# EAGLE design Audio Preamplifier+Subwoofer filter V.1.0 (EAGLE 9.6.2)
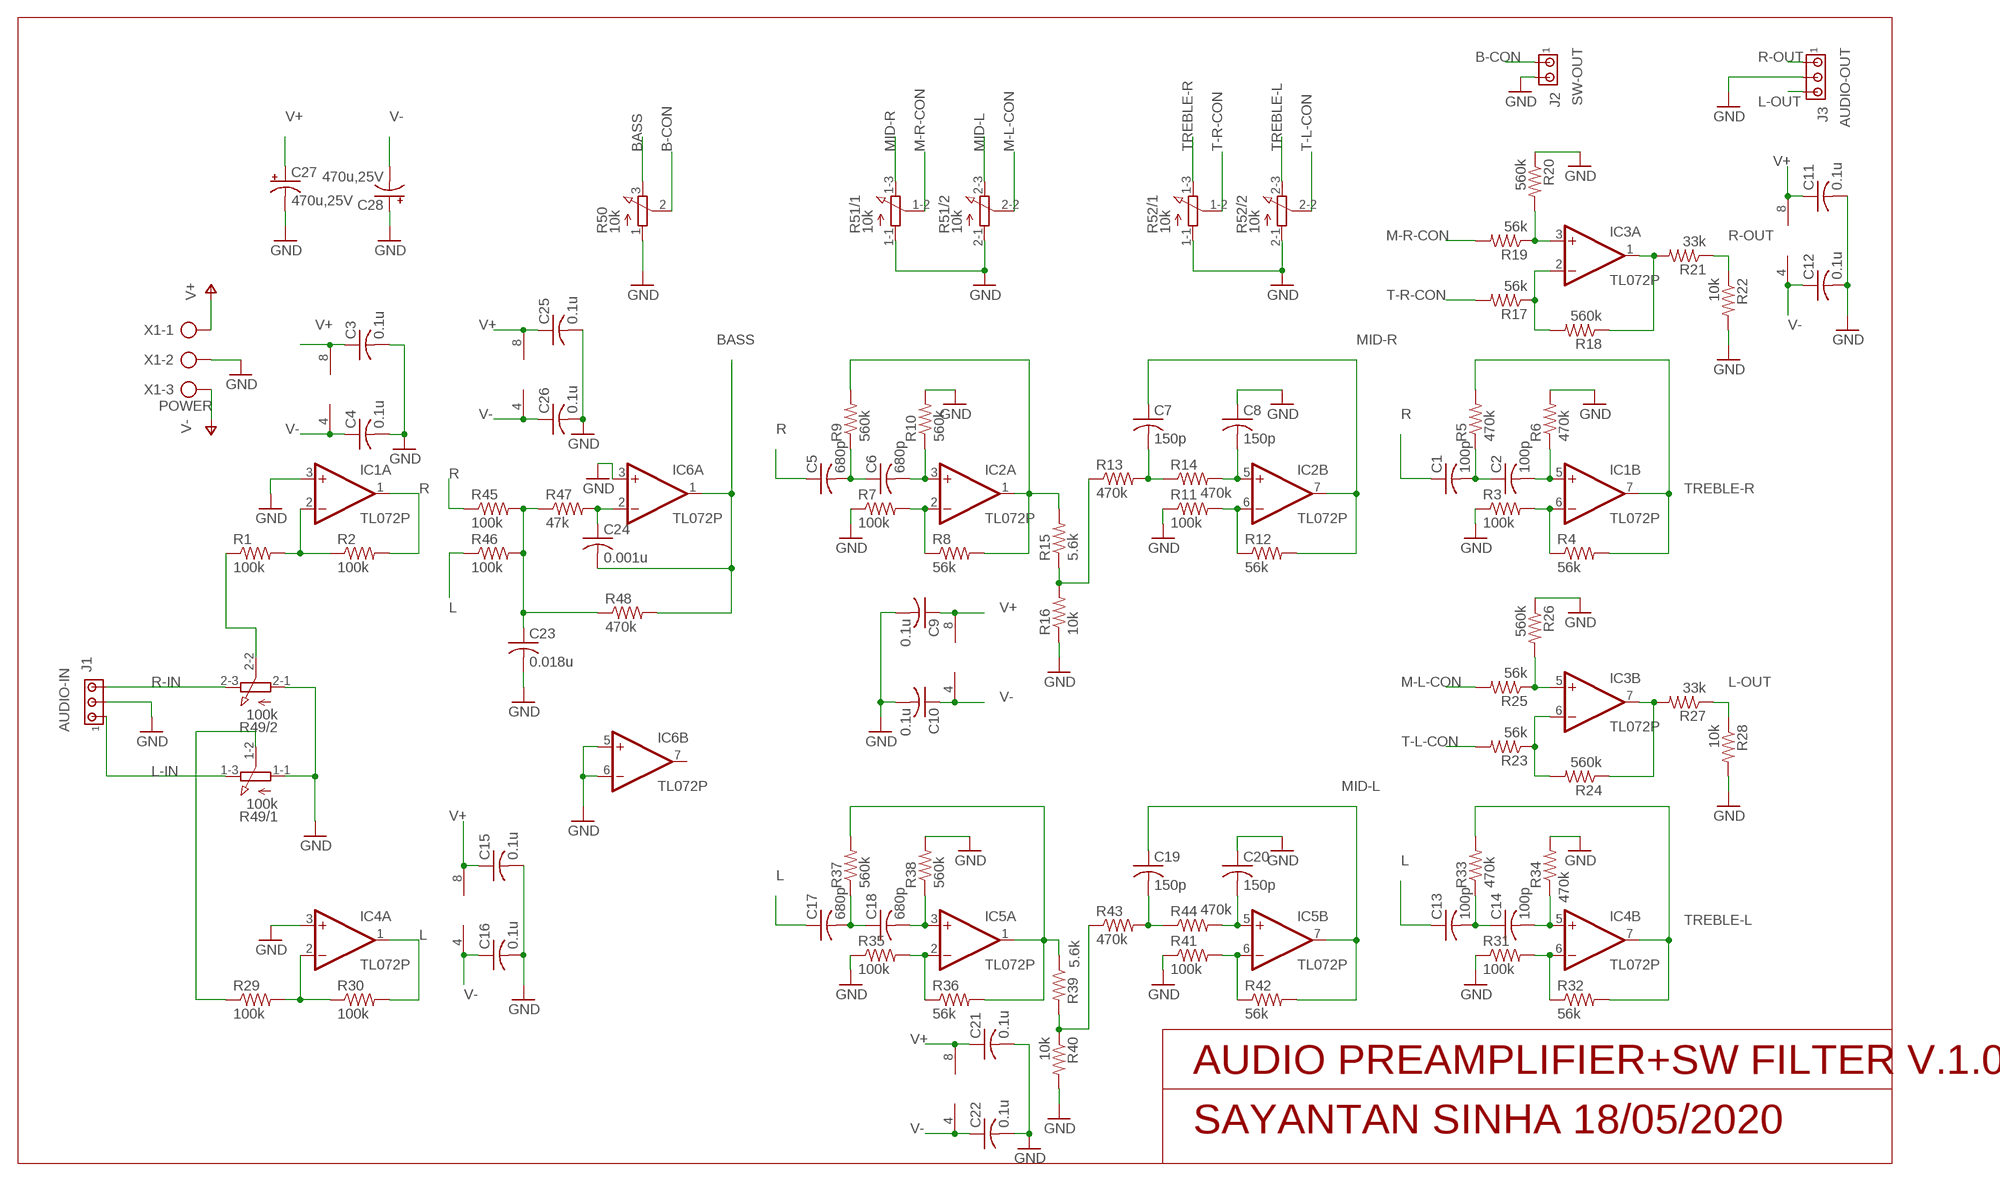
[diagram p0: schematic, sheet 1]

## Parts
C1  100p  C-US025-025X050  [C025-025X050]
C2  100p  C-US025-025X050  [C025-025X050]
C3  0.1u  C-US025-025X050  [C025-025X050]
C4  0.1u  C-US025-025X050  [C025-025X050]
C5  680p  C-US025-025X050  [C025-025X050]
C6  680p  C-US025-025X050  [C025-025X050]
C7  150p  C-US025-025X050  [C025-025X050]
C8  150p  C-US025-025X050  [C025-025X050]
C9  0.1u  C-US025-025X050  [C025-025X050]
C10  0.1u  C-US025-025X050  [C025-025X050]
C11  0.1u  C-US025-025X050  [C025-025X050]
C12  0.1u  C-US025-025X050  [C025-025X050]
C13  100p  C-US025-025X050  [C025-025X050]
C14  100p  C-US025-025X050  [C025-025X050]
C15  0.1u  C-US025-025X050  [C025-025X050]
C16  0.1u  C-US025-025X050  [C025-025X050]
C17  680p  C-US025-025X050  [C025-025X050]
C18  680p  C-US025-025X050  [C025-025X050]
C19  150p  C-US025-025X050  [C025-025X050]
C20  150p  C-US025-025X050  [C025-025X050]
C21  0.1u  C-US025-025X050  [C025-025X050]
C22  0.1u  C-US025-025X050  [C025-025X050]
C23  0.018u  C-US025-025X050  [C025-025X050]
C24  0.001u  C-US025-025X050  [C025-025X050]
C25  0.1u  C-US025-025X050  [C025-025X050]
C26  0.1u  C-US025-025X050  [C025-025X050]
C27  470u,25V  CPOL-USE5-10.5  [E5-10,5]
C28  470u,25V  CPOL-USE5-10.5  [E5-10,5]
IC1  TL072P  [DIL08]
IC2  TL072P  [DIL08]
IC3  TL072P  [DIL08]
IC4  TL072P  [DIL08]
IC5  TL072P  [DIL08]
IC6  TL072P  [DIL08]
J1  AUDIO-IN  MTA03-100  [10X03MTA]
J2  SW-OUT  MTA02-100  [10X02MTA]
J3  AUDIO-OUT  MTA03-100  [10X03MTA]
R1  100k  R-US_0207/10  [0207/10]
R2  100k  R-US_0207/10  [0207/10]
R3  100k  R-US_0207/10  [0207/10]
R4  56k  R-US_0207/10  [0207/10]
R5  470k  R-US_0207/10  [0207/10]
R6  470k  R-US_0207/10  [0207/10]
R7  100k  R-US_0207/10  [0207/10]
R8  56k  R-US_0207/10  [0207/10]
R9  560k  R-US_0207/10  [0207/10]
R10  560k  R-US_0207/10  [0207/10]
R11  100k  R-US_0207/10  [0207/10]
R12  56k  R-US_0207/10  [0207/10]
R13  470k  R-US_0207/10  [0207/10]
R14  470k  R-US_0207/10  [0207/10]
R15  5.6k  R-US_0207/10  [0207/10]
R16  10k  R-US_0207/10  [0207/10]
R17  56k  R-US_0207/10  [0207/10]
R18  560k  R-US_0207/10  [0207/10]
R19  56k  R-US_0207/10  [0207/10]
R20  560k  R-US_0207/10  [0207/10]
R21  33k  R-US_0207/10  [0207/10]
R22  10k  R-US_0207/10  [0207/10]
R23  56k  R-US_0207/10  [0207/10]
R24  560k  R-US_0207/10  [0207/10]
R25  56k  R-US_0207/10  [0207/10]
R26  560k  R-US_0207/10  [0207/10]
R27  33k  R-US_0207/10  [0207/10]
R28  10k  R-US_0207/10  [0207/10]
R29  100k  R-US_0207/10  [0207/10]
R30  100k  R-US_0207/10  [0207/10]
R31  100k  R-US_0207/10  [0207/10]
R32  56k  R-US_0207/10  [0207/10]
R33  470k  R-US_0207/10  [0207/10]
R34  470k  R-US_0207/10  [0207/10]
R35  100k  R-US_0207/10  [0207/10]
R36  56k  R-US_0207/10  [0207/10]
R37  560k  R-US_0207/10  [0207/10]
R38  560k  R-US_0207/10  [0207/10]
R39  5.6k  R-US_0207/10  [0207/10]
R40  10k  R-US_0207/10  [0207/10]
R41  100k  R-US_0207/10  [0207/10]
R42  56k  R-US_0207/10  [0207/10]
R43  470k  R-US_0207/10  [0207/10]
R44  470k  R-US_0207/10  [0207/10]
R45  100k  R-US_0207/10  [0207/10]
R46  100k  R-US_0207/10  [0207/10]
R47  47k  R-US_0207/10  [0207/10]
R48  470k  R-US_0207/10  [0207/10]
R49  100k  3RP/1610G  [3RP/1610G]
R50  10k  3RP/1610N  [3RP/1610N]
R51  10k  3RP/1610G  [3RP/1610G]
R52  10k  3RP/1610G  [3RP/1610G]
X1  POWER  AK500/3-H  [AK500/3-H]

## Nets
B-CON: J2.1 R50.2(S)
BASS: C24.2 IC6.1(A:OUT) R48.2 R50.3(E)
GND: C3.2 C4.2 C8.1 C9.2 C10.2 C11.2 C12.2 C15.2 C16.2 C20.1 C21.2 C22.2 C23.2 C25.2 C26.2 C27.- C28.+ IC1.3(A:+IN) IC4.3(A:+IN) IC6.3(A:+IN) IC6.5(B:+IN) IC6.6(B:-IN) J1.2 J2.2 J3.2 R3.1 R6.2 R7.1 R10.2 R11.1 R16.1 R20.1 R22.2 R26.1 R28.2 R31.1 R34.2 R35.1 R38.2 R40.2 R41.1 R49.1-1(/1:A) R49.2-1(/2:A) R50.1(A) R51.1-1(/1:A) R51.2-1(/2:A) R52.1-1(/1:A) R52.2-1(/2:A) X1.2
L: C13.1 C17.1 IC4.1(A:OUT) R30.2 R46.1
L-IN: J1.1 R49.1-3(/1:E)
L-OUT: J3.3 R27.1 R28.1
M-L-CON: R25.2 R51.2-2(/2:S)
M-R-CON: R19.2 R51.1-2(/1:S)
MID-L: C19.1 IC5.7(B:OUT) R42.2 R51.2-3(/2:E)
MID-R: C7.1 IC2.7(B:OUT) R12.2 R51.1-3(/1:E)
N$1: C23.1 R45.2 R46.2 R47.1 R48.1
N$3: C24.1 IC6.2(A:-IN) R47.2
N$4: R1.1 R49.2-2(/2:S)
N$5: IC2.2(A:-IN) R7.2 R8.1
N$6: IC2.1(A:OUT) R8.2 R9.2 R15.2
N$7: IC2.6(B:-IN) R11.2 R12.1
N$8: R29.1 R49.1-2(/1:S)
N$9: IC1.6(B:-IN) R3.2 R4.1
N$10: IC1.2(A:-IN) R1.2 R2.1
N$11: IC3.6(B:-IN) R23.1 R24.2
N$12: IC3.7(B:OUT) R24.1 R27.2
N$13: IC4.2(A:-IN) R29.2 R30.1
N$14: IC4.6(B:-IN) R31.2 R32.1
N$16: IC5.6(B:-IN) R41.2 R42.1
N$18: IC5.1(A:OUT) R36.2 R37.2 R39.1
N$19: R39.2 R40.1 R43.1
N$20: IC5.2(A:-IN) R35.2 R36.1
N$23: IC3.5(B:+IN) R25.1 R26.2
N$25: IC3.2(A:-IN) R17.1 R18.2
N$26: IC3.3(A:+IN) R19.1 R20.2
N$28: IC3.1(A:OUT) R18.1 R21.2
N$30: R13.1 R15.1 R16.2
N$33: C5.2 C6.1 R9.1
N$34: C6.2 IC2.3(A:+IN) R10.1
N$35: C7.2 R13.2 R14.1
N$36: C8.2 IC2.5(B:+IN) R14.2
N$37: C1.2 C2.1 R5.1
N$38: C2.2 IC1.5(B:+IN) R6.1
N$44: C14.2 IC4.5(B:+IN) R34.1
N$45: C13.2 C14.1 R33.1
N$46: C20.2 IC5.5(B:+IN) R44.2
N$47: C19.2 R43.2 R44.1
N$49: C17.2 C18.1 R37.1
N$51: C18.2 IC5.3(A:+IN) R38.1
R: C1.1 C5.1 IC1.1(A:OUT) R2.2 R45.1
R-IN: J1.3 R49.2-3(/2:E)
R-OUT: J3.1 R21.1 R22.1
T-L-CON: R23.2 R52.2-2(/2:S)
T-R-CON: R17.2 R52.1-2(/1:S)
TREBLE-L: IC4.7(B:OUT) R32.2 R33.2 R52.2-3(/2:E)
TREBLE-R: IC1.7(B:OUT) R4.2 R5.2 R52.1-3(/1:E)
V+: C3.1 C9.1 C11.1 C15.1 C21.1 C25.1 C27.+ IC1.8(P:V+) IC2.8(P:V+) IC3.8(P:V+) IC4.8(P:V+) IC5.8(P:V+) IC6.8(P:V+) X1.1
V-: C4.1 C10.1 C12.1 C16.1 C22.1 C26.1 C28.- IC1.4(P:V-) IC2.4(P:V-) IC3.4(P:V-) IC4.4(P:V-) IC5.4(P:V-) IC6.4(P:V-) X1.3
Unconnected: IC6.7(B:OUT)

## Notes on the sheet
- AUDIO PREAMPLIFIER+SW FILTER V.1.0
- SAYANTAN SINHA 18/05/2020

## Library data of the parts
C1-C26 = rcl:C-US: CAPACITOR, American symbol; SPICEPREFIX: C
C27 C28 = rcl:CPOL-US: POLARIZED CAPACITOR, American symbol; SPICEPREFIX: C
IC1-IC6 = linear:TL072: OP AMP
J1 J3 = con-amp:MTA03-100: AMP connector
J2 = con-amp:MTA02-100: AMP connector
R1-R48 = rcl:R-US_: RESISTOR, American symbol; SPICEPREFIX: R
R49 R51 R52 = pot:3RP/1610G: 16mm Potentiometer two level Source: http://www.alphapotentiometers.net/html/16mm_pot_2.html
R50 = pot:3RP/1610N: 16mm Potentiometer one level Source: http://www.alphapotentiometers.net/html/16mm_pot_2.html
X1 = con-ptr500:AK500/3-H: CONNECTOR Aug. 2004 / PTR Meßtechnik: Die Bezeichnung der Serie AK505 wurde geändert. Es handelt sich hierbei um AK500 in horizontaler Ausführung.; OC_FARNELL: unknown; OC_NEWARK: unknown

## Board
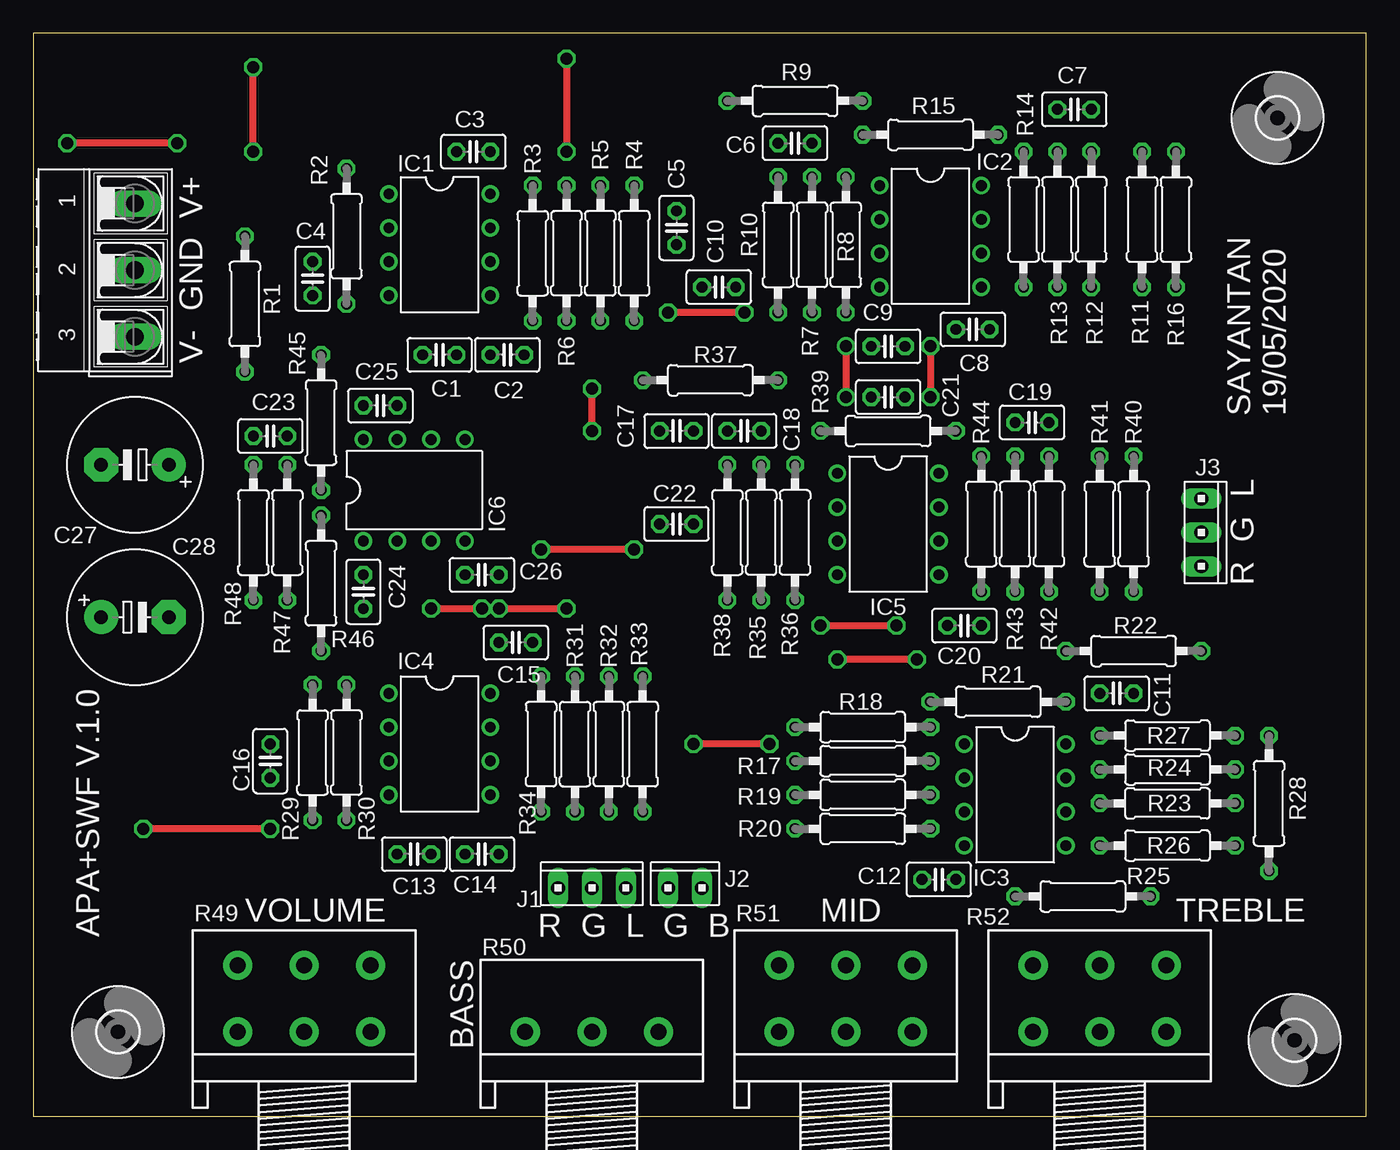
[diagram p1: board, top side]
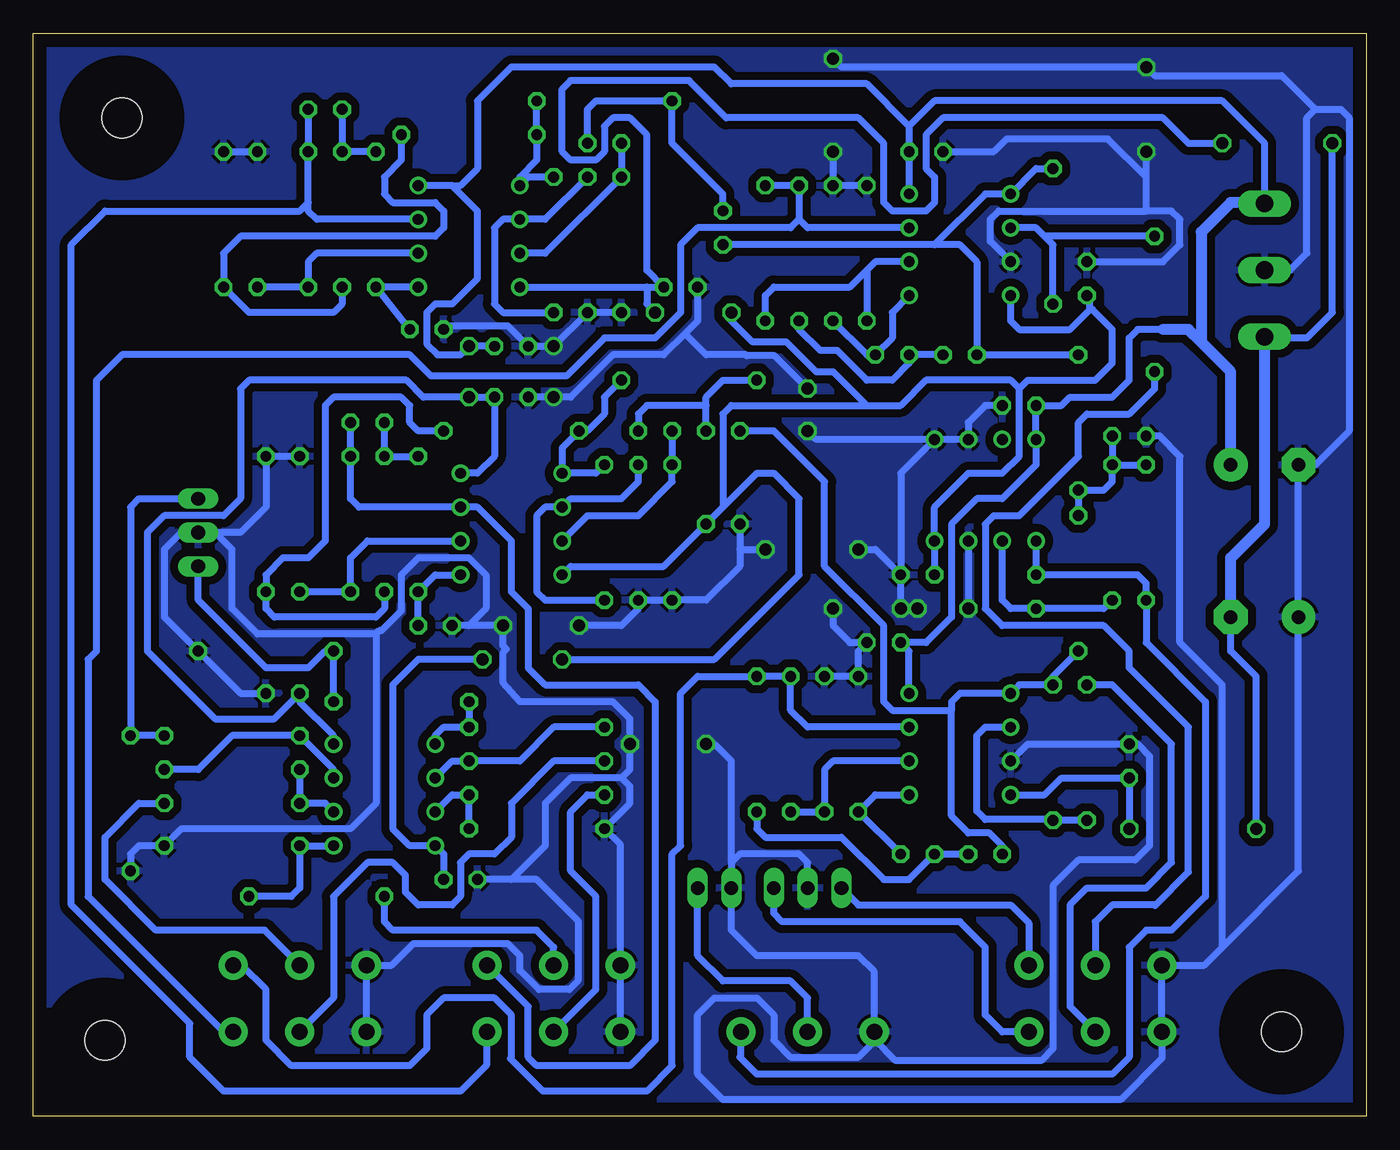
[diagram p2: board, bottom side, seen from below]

Size 100 x 81.27 mm. Coordinates in mm from the lower left corner, seen from the top.
Outline: 0,0 100,0 100,81.27 0,81.27 0,0
Copper layers (1*16): Top 0.035mm / dielectric 1.5mm / Bottom 0.035mm
Design rules "default *": minimum track width 6mil, minimum drill 0.35mm, track to track 20mil, track to pad 10mil, pad to pad 6mil, via to via 6mil, smd to smd 6mil, copper to edge 40mil, drill to drill 6mil, minimum pad ring 10mil, minimum via ring 8mil, stop-mask expansion 4mil, vias tented up to drill 0mil, thermal gap 10mil

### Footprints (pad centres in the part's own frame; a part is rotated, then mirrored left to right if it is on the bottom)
C025-025X050 = drill 0.813 octagon: 1 -1.27,0; 2 1.27,0
E5-10,5 = drill 1.016 pad 2.54: + -2.54,0 | drill 1.016 pad 2.54 octagon: - 2.54,0
DIL08 = drill 0.813 pad 1.27: 1 -3.81,-3.81; 2 -1.27,-3.81; 3 1.27,-3.81; 4 3.81,-3.81; 5 3.81,3.81; 6 1.27,3.81; 7 -1.27,3.81; 8 -3.81,3.81
10X03MTA = drill 1.016 long: 1 2.54,0; 2 0,0; 3 -2.54,0
10X02MTA = drill 1.016 long: 1 1.27,0; 2 -1.27,0
0207/10 = drill 0.813 octagon: 1 -5.08,0; 2 5.08,0
3RP/1610G = drill 1.2 pad 2.184: 1-1 -5,0; 1-2 0,0; 1-3 5,0; 2-1 -5,5; 2-2 0,5; 2-3 5,5
3RP/1610N = drill 1.2 pad 2.184: 1 -5,0; 2 0,0; 3 5,0
3,0 = hole 3: 0,0
AK500/3-H = drill 1.321 long: 1 -5.004,0; 2 0,0; 3 5.004,0

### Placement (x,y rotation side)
C1  30.48,57.15 0 top
C2  35.56,57.15 0 top
C3  33.02,72.39 180 top
C4  20.95,62.87 90 top
C5  48.26,66.68 90 top
C6  57.15,73.03 180 top
C7  78.11,75.57 180 top
C8  70.48,59.05 0 top
C9  64.14,57.78 180 top
C10  51.44,62.23 180 top
C11  81.28,31.75 0 top
C12  67.94,17.78 180 top
C13  28.57,19.68 0 top
C14  33.66,19.68 0 top
C15  36.2,35.56 0 top
C16  17.78,26.67 90 top
C17  48.26,51.44 0 top
C18  53.34,51.44 180 top
C19  74.93,52.07 180 top
C20  69.85,36.83 0 top
C21  64.14,53.98 180 top
C22  48.26,44.45 180 top
C23  17.78,51.05 180 top
C24  24.77,39.37 90 top
C25  26.04,53.34 0 top
C26  33.66,40.64 0 top
C27  7.62,48.89 180 top
C28  7.62,37.46 0 top
IC1  30.48,65.41 270 top
IC2  67.31,66.04 270 top
IC3  73.66,24.13 270 top
IC4  30.48,27.94 270 top
IC5  64.14,44.45 270 top
IC6  28.57,46.99 0 top
J1  41.91,17.14 0 top
J2  48.9,17.14 0 top
J3  87.63,43.81 270 top
R1  15.88,60.96 90 top
R2  23.5,66.04 90 top
R3  37.47,64.77 270 top
R4  45.09,64.77 90 top
R5  42.55,64.77 90 top
R6  40.01,64.77 90 top
R7  58.42,65.41 90 top
R8  60.96,65.41 90 top
R9  57.15,76.2 0 top
R10  55.88,65.41 270 top
R11  83.19,67.31 270 top
R12  79.38,67.31 90 top
R13  76.83,67.31 90 top
R14  74.3,67.31 270 top
R15  67.31,73.66 180 top
R16  85.72,67.31 270 top
R17  62.23,26.67 180 top
R18  62.23,29.21 180 top
R19  62.23,24.13 180 top
R20  62.23,21.59 0 top
R21  72.39,31.11 180 top
R22  82.55,34.92 0 top
R23  85.09,23.49 0 top
R24  85.09,26.04 180 top
R25  78.74,16.51 180 top
R26  85.09,20.32 180 top
R27  85.09,28.57 180 top
R28  92.71,23.49 270 top
R29  20.95,27.3 270 top
R30  23.5,27.3 90 top
R31  40.64,27.94 270 top
R32  43.18,27.94 90 top
R33  45.72,27.94 90 top
R34  38.1,27.94 90 top
R35  54.61,43.81 90 top
R36  57.15,43.81 90 top
R37  50.8,55.24 0 top
R38  52.07,43.81 270 top
R39  64.14,51.44 0 top
R40  82.55,44.45 90 top
R41  80.01,44.45 270 top
R42  76.2,44.45 90 top
R43  73.66,44.45 90 top
R44  71.12,44.45 270 top
R45  21.59,52.07 270 top
R46  21.59,40.01 90 top
R47  19.05,43.81 270 top
R48  16.51,43.81 270 top
R49  20.32,6.35 0 top
R50  41.91,6.35 0 top
R51  60.96,6.35 0 top
R52  80.01,6.35 0 top
U$1  [3,0]  6.35,6.35 0 top
U$2  [3,0]  94.61,5.71 0 top
U$3  [3,0]  93.34,74.93 0 top
X1  7.62,63.5 270 top

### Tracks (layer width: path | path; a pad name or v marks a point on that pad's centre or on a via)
B-CON
  Bottom 0.508: R50.2 41.91,8.89 43.18,10.16 48.26,10.16 50.16,12.07 J2.1
BASS
  Bottom 0.508: IC6.1 C24.2 17.14,40.64 16.51,40.01 R48.2 16.51,35.56 12.06,31.11 12.06,16.51 14.61,13.97 16.51,13.97 17.78,12.7 17.78,4.45 19.05,3.17 45.72,3.17 46.99,4.45 46.91,4.53 R50.3
GND  (via drill 0.9)
  Top 0.508: v59.05,36.83 v64.77,36.83 | v55.24,27.94 v49.53,27.94 | v45.09,42.55 v38.1,42.55 | v34.92,38.1 v40.01,38.1 | v60.96,57.78 v60.96,53.98 | v16.51,72.39 v16.51,78.74 | v40.01,79.38 v40.01,72.39 | v41.91,51.44 v41.91,54.61 | v29.84,38.1 v33.66,38.1
  Bottom 0.508: R3.1 R6.2 v40.01,72.39 | R10.2 R7.1 v60.96,57.78 C9.2 64.39,59.31 68.83,59.31 68.9,59.37 C8.1 | R16.1 R11.1 | IC6.5 IC6.6 29.84,52.07 28.57,53.34 C25.2 | R31.1 R34.2 38.1,34.92 C15.2 38.73,35.56 40.01,36.83 v40.01,38.1 | R41.1 R40.2 82.55,45.72 84.45,43.81 86.36,43.81 | R52.1-1 R52.2-1 73.11,11.35 71.5,12.95 64.39,12.95 63.5,12.07 63.5,10.96 62.06,9.53 59.77,9.53 59.14,10.16 59.14,14.69 62.23,17.78 64.14,17.78 | R51.1-1 R51.2-1 55.96,20.4 R20.1 55.24,23.49 55.24,24.77 55.88,25.4 | 64.14,17.78 61.59,20.32 61.59,23.49 59.69,25.4 55.88,25.4 | 64.14,17.78 C12.2 | 55.88,25.4 55.24,26.04 v55.24,27.94 55.24,29.84 56.52,31.11 63.5,31.11 64.75,32.53 64.75,34.81 64.52,35.05 64.77,35.31 v64.77,36.83 67.31,36.83 | 74.3,36.2 74.04,36.45 73.87,36.45 72.39,37.93 72.39,40.64 71.12,41.91 67.31,41.91 66.04,40.64 66.04,38.1 67.31,36.83 | 74.3,36.2 83.19,36.2 85.09,38.1 85.09,42.55 86.36,43.81 | 86.36,43.81 J3.2 88.9,43.81 90.17,42.55 90.17,37.46 R22.2 84.45,31.75 C11.2 | IC1.3 28.19,65.66 28.19,67.31 27.56,67.95 16.51,67.95 | C4.2 15.24,64.14 13.97,65.41 13.97,67.31 14.61,67.95 16.51,67.95 | C3.2 27.94,72.39 26.99,73.34 19.37,73.34 16.51,70.48 | 16.51,67.95 16.51,70.48 | J1.2 41.91,19.05 42.55,19.68 46.99,19.68 47.62,19.05 | 47.62,19.05 J2.2 47.62,13.97 45.72,12.07 38.1,12.07 36.91,10.88 R50.1 36.91,5.79 36.83,5.71 | 47.62,19.05 47.62,26.67 48.9,27.94 v49.53,27.94 | IC4.3 25.4,27.94 C16.2 17.14,27.94 16.26,27.05 16.26,20.32 17.34,19.24 21.59,19.24 23.5,17.34 23.5,5.08 24.38,4.19 35.31,4.19 36.83,5.71 | IC6.5 34.92,48.26 C26.2 | C22.2 46.99,42.55 | 46.99,42.55 46.99,41.27 49.53,38.73 R38.2 R35.1 54.61,38.1 55.88,36.83 v59.05,36.83
  Bottom 0.508: 67.31,36.83 C20.1 | R28.2 92.71,19.68 92.08,20.32 R26.1 88.9,21.59 76.2,21.59 74.3,23.49 74.3,36.2 | 10.79,12.7 12.14,11.35 R49.2-1 R49.1-1 15.32,4.37 18.41,1.27 48.26,1.27 50.16,3.17 50.16,7.62 48.9,8.89 45.72,8.89 44.45,7.62 44.45,5.71 43.18,4.45 38.1,4.45 36.83,5.71 | 10.79,12.7 5.08,18.41 C28.+ C27.- 3.81,48.89 1.27,51.44 1.27,74.93 1.91,75.57 3.81,75.57 | 46.99,42.55 v45.09,42.55 | v38.1,42.55 36.83,42.55 C26.2 | 10.79,12.7 10.79,32.38 13.97,35.56 13.97,49.53 15.49,51.05 C23.2 | C26.2 v34.92,38.1 v33.66,38.1 | IC6.3 v29.84,38.1 | C21.2 v60.96,53.98 59.69,53.98 56.52,57.15 52.7,57.15 51.12,58.74 | C10.2 50.16,59.69 51.12,58.74 | X1.2 5.71,63.5 4.45,64.77 4.45,74.93 3.81,75.57 | 16.51,70.48 v16.51,72.39 | 3.81,75.57 6.35,78.11 15.88,78.11 v16.51,78.74 39.37,78.74 v40.01,79.38 | v41.91,51.44 41.27,50.8 IC6.5 | v41.91,54.61 44.39,57.09 46.46,57.09 46.52,57.15 49.53,57.15 51.12,58.74
  pour Bottom (isolate 0.61): 0,81.28 99.69,81.28 99.69,0 0,0
L
  Bottom 0.508: R46.1 23.5,33.02 R30.2 26.04,32.38 IC4.1 30.48,31.75 31.11,31.11 31.11,30.48 | C13.1 27.3,20.32 28.26,21.27 29.84,21.27 31.11,22.54 31.11,30.48 | 31.11,30.48 35.56,30.48 36.2,31.11 36.2,36.83 40.64,41.27 40.64,47.62 44.45,51.44 C17.1
L-IN
  Bottom 0.508: R49.1-3 27.3,6.35 28.57,7.62 28.57,12.7 30.48,14.61 43.81,14.61 44.45,15.24 J1.1
L-OUT
  Bottom 0.508: R27.1 R28.1 92.71,45.72 92.08,46.35 J3.3
M-L-CON
  Bottom 0.508: R51.2-2 60.96,12.7 62.23,13.97 73.03,13.97 73.66,14.61 R25.2
M-R-CON
  Bottom 0.508: R19.2 58.42,24.13 59.69,22.86 59.69,18.41 57.78,16.51 57.78,9.53 R51.1-2
MID-L
  Bottom 0.508: C19.1 R42.2 76.2,46.35 75.56,45.72 IC5.7 66.67,45.72 64.14,43.18 64.14,39.37 62.87,38.1 62.87,33.66 61.59,32.38 54.61,32.38 53.34,31.11 53.34,5.71 55.24,3.81 62.23,3.81 62.87,4.45 62.87,8.25 R51.2-3
MID-R
  Bottom 0.508: C7.1 R12.2 79.38,68.58 | R51.1-3 65.96,3.89 67.94,1.91 85.72,1.91 88.27,4.45 88.27,6.99 97.16,15.88 97.16,65.41 94.61,67.95 80.01,67.95 79.38,68.58 | IC2.7 78.74,67.31 79.38,67.95 79.38,68.58
N$1
  Bottom 0.508: C23.1 R47.1 | R47.1 R48.1 | R46.2 R45.2 19.68,46.99 19.05,47.62 R47.1
N$3
  Bottom 0.508: R47.2 19.68,38.1 C24.1 26.67,38.1 27.3,38.73 IC6.2
N$4
  Bottom 0.508: R49.2-2 20.32,14.61 19.05,15.88 15.88,15.88 15.84,15.84 13.34,18.34 13.34,29.21 17.78,33.66 17.78,34.92 19.68,36.83 27.3,36.83 28.57,38.1 28.57,44.45 27.94,45.09 26.04,45.09 21.59,49.53 21.59,52.07 20.95,52.7 17.78,52.7 15.88,54.61 R1.1
N$5
  Bottom 0.508: R8.1 64.77,60.32 65.41,60.96 65.41,66.68 64.77,67.31 IC2.2 61.59,67.31 R7.2
N$6
  Bottom 0.508: R8.2 62.87,70.48 IC2.1 63.5,70.48 62.23,71.76 R15.2 R9.2
N$7
  Bottom 0.508: R11.2 R12.1 79.38,64.14 78.74,64.77 IC2.6
N$8
  Bottom 0.508: R49.1-2 22.23,8.25 22.23,15.88 20.95,17.14 16.51,17.14 14.61,19.05 14.61,27.94 19.05,32.38 R29.1
N$9
  Bottom 0.508: IC1.6 36.83,64.14 37.47,63.5 | 37.47,63.5 R3.2 | R4.1 45.09,61.59 44.45,62.23 38.73,62.23 37.47,63.5
N$10
  Bottom 0.508: R2.1 23.5,65.41 24.13,66.04 | IC1.2 24.77,66.68 24.13,66.04 | R1.2 24.13,66.04
N$11
  Bottom 0.508: IC3.6 78.11,23.49 R23.1 R24.2
N$12
  Bottom 0.508: IC3.7 77.47,26.04 R27.2 85.09,28.57 87.63,26.04 R24.1
N$13
  Bottom 0.508: R29.2 R30.1 23.56,22.29 28.57,22.29 29.21,22.92 29.21,28.57 28.57,29.21 IC4.2
N$14
  Bottom 0.508: R32.1 R31.2 40.64,26.04 40.01,26.67 IC4.6
N$16
  Bottom 0.508: IC5.6 74.93,43.18 76.2,41.91 R42.1 R41.2
N$18
  Bottom 0.508: R36.2 57.78,48.26 IC5.1 60.33,50.16 R39.1 58.42,51.44 57.15,52.7 57.15,53.98 R37.2
N$19
  Bottom 0.508: R39.2 71.12,51.44 71.75,52.07 71.75,53.34 72.39,53.98 77.47,53.98 78.11,53.34 78.11,43.18 79.38,41.91 81.28,41.91 82.55,40.64 R40.1 82.55,38.1 81.92,37.46 74.3,37.46 73.66,38.1 R43.1
N$20
  Bottom 0.508: R36.1 61.59,38.73 62.23,39.37 62.23,45.09 61.59,45.72 IC5.2 59.69,46.35 55.88,46.35 54.61,47.62 R35.2
N$23
  Bottom 0.508: R25.1 80.64,16.51 80.01,17.14 R26.2 IC3.5
N$25
  Bottom 0.508: IC3.2 68.58,26.67 R17.1 63.5,26.67 60.96,29.21 R18.2
N$26
  Bottom 0.508: IC3.3 68.58,24.13 R19.1 R20.2
N$28
  Bottom 0.508: IC3.1 69.85,28.57 69.22,29.21 R18.1 R21.2
N$30
  Bottom 0.508: R13.1 76.83,60.96 77.47,60.32 83.82,60.32 R16.2 85.72,64.77 84.45,66.04 69.85,66.04 69.22,66.68 69.22,67.95 69.85,68.58 73.03,68.58 73.66,69.22 73.66,70.48 72.39,71.76 R15.1
N$33
  Bottom 0.508: C5.2 48.26,69.22 52.07,73.03 R9.1 57.78,76.2 58.42,75.57 C6.1
N$34
  Bottom 0.508: C6.2 R10.1 61.59,64.77 IC2.3
N$35
  Bottom 0.508: R14.1 R13.2 C7.2
N$36
  Bottom 0.508: IC2.5 R14.2 C8.2
N$37
  Bottom 0.508: C1.2 C2.1 34.29,56.52 35.56,55.24 37.47,55.24 39.69,57.47 40.96,57.47 42.55,59.05 R5.1
N$38
  Bottom 0.508: IC1.5 35.56,60.32 35.56,58.42 C2.2 37.47,57.15 R6.1
N$44
  Bottom 0.508: IC4.5 36.83,24.13 R34.1 C14.2
N$45
  Bottom 0.508: C13.2 C14.1 34.29,17.78 36.2,17.78 39.37,20.95 45.09,20.95 45.72,21.59 R33.1
N$46
  Bottom 0.508: IC5.5 69.85,40.64 R44.2 C20.2
N$47
  Bottom 0.508: C19.2 R43.2 R44.1
N$49
  Bottom 0.508: C17.2 49.53,53.34 | C18.1 54.61,52.7 53.98,53.34 49.53,53.34 | 49.53,53.34 49.53,53.98 48.26,55.24 R37.1
N$51
  Bottom 0.508: C18.2 R38.1 52.07,47.62 54.61,45.09 58.42,45.09 IC5.3
R
  Bottom 0.508: R45.1 C1.1 29.21,64.14 30.48,65.41 32.38,65.41 | R2.2 24.77,71.12 IC1.1 28.57,69.22 32.38,65.41 | 32.38,65.41 C5.1
R-IN
  Bottom 0.508: J1.3 38.1,15.88 26.67,15.88 25.32,14.52 R49.2-3
R-OUT
  Bottom 0.508: R21.1 R22.1 78.11,34.92 79.38,33.66 82.55,33.66 87.63,38.73 J3.1
T-L-CON
  Bottom 0.508: R52.2-2 82.63,13.97 90.81,13.97 94.61,17.78 94.61,20.95 92.08,23.49 R23.2
T-R-CON
  Bottom 0.508: R52.1-2 77.47,8.89 77.47,16.51 74.93,19.05 73.03,19.05 72.07,18.1 72.07,16.83 71.12,15.88 68.58,15.88 67.94,16.51 67.94,19.05 67.31,19.68 65.41,19.68 64.14,20.95 64.14,23.49 60.96,26.67 R17.2
TREBLE-L
  Bottom 0.508: IC4.7 41.91,29.21 43.18,30.48 R32.2 R33.2 50.16,33.02 51.44,31.75 51.44,20.32 52.07,19.68 52.07,3.81 53.98,1.91 61.76,1.91 64.22,4.36 64.14,4.45 64.14,7.62 65.41,8.89 69.22,8.89 70.48,7.62 70.48,5.08 71.75,3.81 80.64,3.81 82.55,5.71 82.55,9.53 84.38,11.35 R52.2-3
TREBLE-R
  Bottom 0.508: IC1.7 41.91,66.68 42.55,67.31 | R4.2 R5.2 42.55,67.31 | 42.55,67.31 43.18,66.68 50.16,66.68 51.44,65.41 51.44,60.32 53.34,58.42 57.15,58.42 60.01,55.56 70.17,55.56 71.75,57.15 93.34,57.15 95.25,55.24 95.25,34.92 95.89,34.29 95.89,16.51 85.72,6.35 R52.1-3
V+  (via drill 0.9)
  Top 0.508: v67.31,57.78 v67.31,53.98
  Bottom 0.508: IC1.8 C3.1 34.29,74.3 | 68.58,69.85 66.67,67.95 66.67,62.87 68.58,60.96 69.85,60.96 70.48,60.32 70.48,57.95 69.68,57.15 67.94,57.15 v67.31,57.78 C9.1 | 68.58,69.85 IC2.8 | IC3.8 77.47,28.57 80.01,31.11 C11.1 81.92,29.84 86.36,29.84 91.44,34.92 91.44,43.81 90.17,45.09 85.72,45.09 84.45,46.35 84.45,54.61 83.82,55.24 72.01,55.24 70.74,53.98 v67.31,53.98 C21.1 65.41,49.53 66.67,48.26 IC5.8 | 34.29,74.3 32.38,76.2 10.79,76.2 7.62,73.03 X1.1 7.54,68.58 | 68.58,69.85 67.94,69.85 66.67,71.12 66.67,76.2 64.14,78.73 48.9,78.73 47.63,77.47 37.47,77.47 34.29,74.3 | 15.24,59.05 17.14,59.05 17.78,58.42 17.78,55.24 19.05,53.98 22.23,53.98 22.86,53.34 C25.1 IC6.8 24.77,48.89 27.3,46.35 29.21,46.35 31.11,44.45 31.11,37.46 33.02,35.56 C15.1 34.29,34.92 IC4.8
  Bottom 0.813: C27.+ 10.16,55.88 12.38,58.1 | X1.1 7.7,68.58 10.16,68.58 12.38,66.36 12.38,58.1 | 12.38,58.1 13.34,59.05 15.24,59.05
V-  (via drill 0.9)
  Top 0.508: v17.78,21.59 v8.26,21.59 | v66.29,34.29 v60.33,34.29 | v10.79,73.03 v2.54,73.03 | v53.34,60.32 v47.62,60.32
  Bottom 0.508: C4.1 20.74,61.51 20.74,60.54 | IC1.4 26.67,59.69 26.04,59.05 22.23,59.05 20.74,60.54 | IC5.4 59.69,41.27 52.7,41.27 C22.1 48.26,45.72 | C26.1 IC6.4 32.38,45.72 29.84,48.26 27.3,48.26 26.04,49.53 26.04,54.61 | C12.1 69.22,19.68 IC3.4 71.75,20.32 73.03,21.59 73.03,32.38 71.12,34.29 v66.29,34.29 | IC2.4 53.98,62.23 | 53.98,62.23 C10.1 53.98,63.5 53.98,73.66 55.24,74.93 56.52,74.93 57.15,74.3 57.15,72.39 57.78,71.76 59.69,71.76 60.33,72.39 60.33,77.09 59.7,77.71 50.8,77.71 48.02,74.93 38.1,74.93 36.2,73.03 36.2,68.58 35.56,67.95 33.02,67.95 32.38,68.58 32.38,70.48 33.02,71.12 33.02,73.66 31.75,74.93 15.24,74.93 13.34,73.03 v10.79,73.03 | 26.04,54.61 25.4,55.24 20.32,55.24 19.05,56.52 19.05,59.05 20.54,60.54 20.74,60.54 | 26.04,54.61 26.67,55.24 33.02,55.24 34.92,53.34 37.47,53.34 | 48.26,45.72 48.26,52.7 47.62,53.34 37.47,53.34 | v17.78,21.59 C16.1 22.86,25.4 24.13,24.13 IC4.4 | v60.33,34.29 48.9,34.29 42.55,40.64 42.55,46.35 44.45,48.26 45.72,48.26 48.26,45.72 | X1.3 7.62,58.42 4.45,58.42 2.54,60.32 v2.54,73.03 | 53.98,62.23 53.98,60.96 v53.34,60.32 | C28.- 10.16,34.92 8.26,33.02 v8.26,21.59 | v47.62,60.32 47.62,59.69 46.04,58.1 43.5,58.1 41.27,55.88 40.01,55.88 37.47,53.34
  Bottom 0.813: C28.- 10.16,41.91 7.62,44.45 7.62,58.42

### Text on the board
tPlace: V- GND V+ | SAYANTAN / 19/05/2020 | R G L | R G L | VOLUME | MID | TREBLE | APA+SWF V.1.0 | G B | BASS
